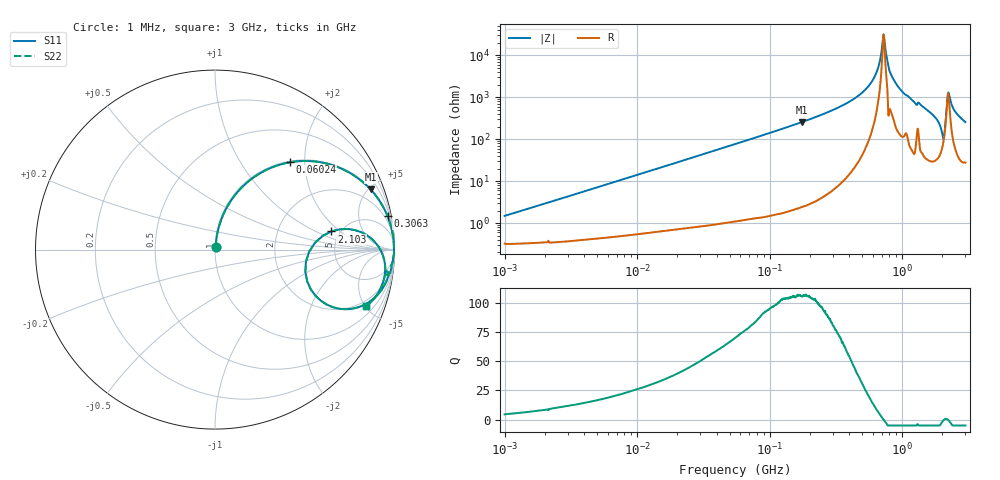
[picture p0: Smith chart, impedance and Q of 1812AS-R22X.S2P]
!s-Parameter Generated by FASTRON Sdn. Bhd.
!FASTRON P/N : 1812AS-R22X
!Keysight Technologies,E4991B,MY54100416,A.01.15
!Date created: Fri Oct 13 15:02:29 2023
!Version  : Rev00 Fri Oct 13 15:02:29 2023
!Data & Calibration Information:
!Freq	S11	S21	S12	S22
!PortZ  Port1:50+j0  Port2:50+j0
!When reading, reference impedance value at option line is always used.
! Remarks : This data is being provided solely for informational purposes.
# Hz S dB R 50
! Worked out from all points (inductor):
!   1601 points, 1 MHz to 3 GHz, reference 50 ohm
!   read as one part in series: L = 231 nH near 1.041 MHz
!   highest Q = 107 at 175.8 MHz (marker M1), where L = 233 nH
!   self-resonance near 724.3 MHz
!   S11 on the Smith chart (normalised r, x): 1 MHz: 1.01, +0.03; 60.24 MHz: 1.02, +1.68; 306.3 MHz: 1, +10; 2.103 GHz: 4.25, +1.52; 3 GHz: 1.55, -5.11
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1000000  -36.56 76.6  -0.03 -0.8  -0.03 -0.8  -36.56 76.6
3804036  -25.32 82.8  -0.05 -3.1  -0.05 -3.1  -25.32 82.8
1.447069e7  -14.08 76.8  -0.23 -11.4  -0.23 -11.4  -14.08 76.8
5.477226e7  -4.39 52.1  -2.06 -37.1  -2.06 -37.1  -4.39 52.1
6.023535e7  -3.89 49.5  -2.38 -39.7  -2.38 -39.7  -3.89 49.5
1.757585e8  -0.64 21.2  -8.85 -68.3  -8.85 -68.3  -0.64 21.2
2.083556e8  -0.45 17.7  -10.35 -71.8  -10.35 -71.8  -0.45 17.7
3.062963e8  -0.18 11.0  -14.37 -78.3  -14.37 -78.3  -0.18 11.0
5.668203e8  -0.03 2.9  -25.96 -84.1  -25.96 -84.1  -0.03 2.9
6.488164e8  -0.03 1.3  -32.86 -81.2  -32.86 -81.2  -0.03 1.3
7.207075e8  -0.03 0.1  -49.49 -18.7  -49.49 -18.7  -0.03 0.1
7.42674e8  -0.03 -0.3  -44.50 57.3  -44.50 57.3  -0.03 -0.3
7.925923e8  -0.02 -1.1  -34.01 84.2  -34.01 84.2  -0.02 -1.1
9.977393e8  -0.07 -4.1  -22.88 81.1  -22.88 81.1  -0.07 -4.1
1.645649e9  -0.37 -13.1  -12.87 72.9  -12.87 72.9  -0.37 -13.1
1.921792e9  -1.39 -22.4  -8.23 56.8  -8.23 56.8  -1.39 -22.4
2.020405e9  -4.19 -24.7  -5.86 30.5  -5.86 30.5  -4.19 -24.7
2.102926e9  -3.66 8.9  -8.73 -16.1  -8.73 -16.1  -3.66 8.9
2.199798e9  -0.81 1.0  -20.87 -10.4  -20.87 -10.4  -0.81 1.0
2.266846e9  -0.48 -3.8  -21.52 48.1  -21.52 48.1  -0.48 -3.8
2.51802e9  -0.44 -12.1  -13.53 70.6  -13.53 70.6  -0.44 -12.1
3e9  -0.92 -20.4  -9.12 63.5  -9.12 63.5  -0.92 -20.4
